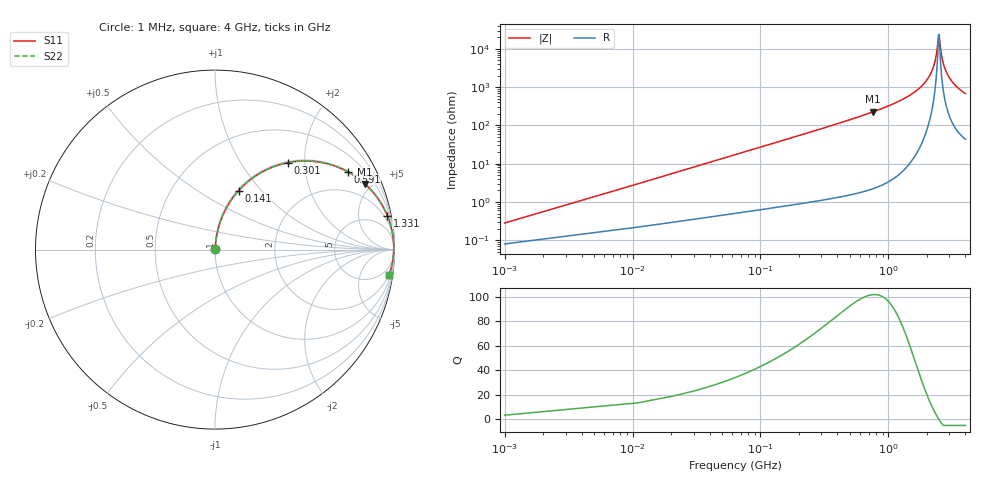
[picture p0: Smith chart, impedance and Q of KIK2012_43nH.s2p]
!version-2
!date-01.2022
!Series
# MHz S RI R 50
!Freq ReS11 ImS11 ReS21 ImS21 ReS12 ImS12 ReS22 ImS22
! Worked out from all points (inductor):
!   401 points, 1 MHz to 4 GHz, reference 50 ohm
!   read as one part in series: L = 43 nH near 21 MHz
!   highest Q = 102 at 761 MHz (marker M1), where L = 47.5 nH
!   self-resonance near 2.481 GHz
!   S11 on the Smith chart (normalised r, x): 1 MHz: 1.00, +0.01; 141 MHz: 1.01, +0.76; 301 MHz: 1.02, +1.65; 591 MHz: 1.03, +3.39; 1.331 GHz: 1, +10; 4 GHz: 2, -14
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1  0.000809 0.0027  0.9992 -0.0027  0.9992 -0.0027  0.000809 0.0027
31  0.0105 0.0826  0.9895 -0.0826  0.9895 -0.0826  0.0105 0.0826
41  0.016 0.1086  0.984 -0.1086  0.984 -0.1086  0.016 0.1086
81  0.0507 0.2068  0.9493 -0.2068  0.9493 -0.2068  0.0507 0.2068
141  0.1323 0.3292  0.8677 -0.3292  0.8677 -0.3292  0.1323 0.3292
301  0.4065 0.4845  0.5935 -0.4845  0.5935 -0.4845  0.4065 0.4845
591  0.7392 0.434  0.2608 -0.434  0.2608 -0.434  0.7392 0.434
671  0.7904 0.4021  0.2096 -0.4021  0.2096 -0.4021  0.7904 0.4021
761  0.835 0.3663  0.165 -0.3663  0.165 -0.3663  0.835 0.3663
1331  0.9598 0.1896  0.0402 -0.1896  0.0402 -0.1896  0.9598 0.1896
1341  0.9608 0.1873  0.0392 -0.1873  0.0392 -0.1873  0.9608 0.1873
2001  0.9926 0.0641  0.00736 -0.0641  0.00736 -0.0641  0.9926 0.0641
2171  0.9949 0.0398  0.0051 -0.0398  0.0051 -0.0398  0.9949 0.0398
2301  0.9957 0.0225  0.00429 -0.0225  0.00429 -0.0225  0.9957 0.0225
2381  0.9959 0.0124  0.00411 -0.0124  0.00411 -0.0124  0.9959 0.0124
2481  0.9958 0.0002  0.00419 -0.0002  0.00419 -0.0002  0.9958 0.0002
2501  0.9958 -0.00217  0.00424 0.00217  0.00424 0.00217  0.9958 -0.00217
2591  0.9954 -0.0126  0.00462 0.0126  0.00462 0.0126  0.9954 -0.0126
2671  0.9949 -0.0216  0.00514 0.0216  0.00514 0.0216  0.9949 -0.0216
2921  0.9923 -0.048  0.00772 0.048  0.00772 0.048  0.9923 -0.048
3341  0.9854 -0.0878  0.0146 0.0878  0.0146 0.0878  0.9854 -0.0878
4000  0.9699 -0.1417  0.0301 0.1417  0.0301 0.1417  0.9699 -0.1417
